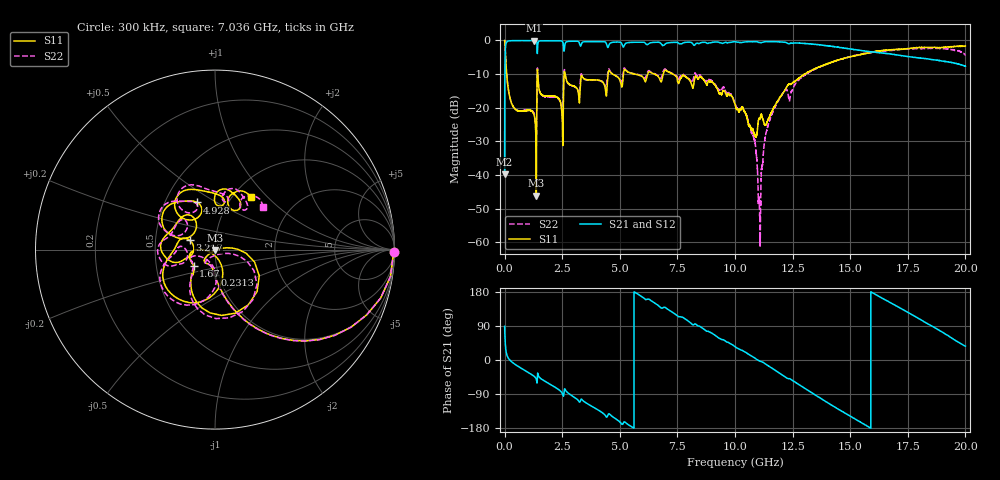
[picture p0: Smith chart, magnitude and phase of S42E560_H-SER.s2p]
!{S42E560}
!Johanson Technology Inc.
!www.johansontechnology.com
!Test Board Conditions:
!Substrate Type  RO4350B
!Substrate Thickness  50 mil
!Substrate Dk  3.66
!TL Type: GCPW
!TL Trace Width  60 mil
!TL Gap  10 mil
!Electrode orientation  Horizontal
!DUT TOPOLOGY	SERIES
!Mounting Pad LxW  14x55 mil
! Created Wed Nov 25 22:20:49 2020
# khz S ma R 50
! 2 Port Network Data from SP1.SP block
! freq  magS11  angS11  magS21  angS21  magS12  angS12  magS22  angS22
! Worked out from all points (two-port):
!   20001 points, 300 kHz to 20 GHz, reference 50 ohm
!   highest |S21| = -0.03 dB at 1.282 GHz (marker M1); lowest = -39.8 dB at 300 kHz (marker M2)
!   |S21| within 3 dB of the highest: 29.19 MHz to 1.413 GHz (1.384 GHz wide, 192 % of centre); 2.586 GHz to 15.52 GHz (12.93 GHz wide, 143 % of centre)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
!   lowest |S11| = -46.1 dB at 1.376 GHz (marker M3), VSWR 1.01, Z = 50.2 - j0.464 ohm
!   |S11| at or under -10 dB: 88.87 MHz to 1.415 GHz (1.326 GHz wide, 176 % of centre); 2.627 GHz to 4.492 GHz (1.865 GHz wide, 52.4 % of centre); 7.299 GHz to 13.01 GHz (5.716 GHz wide, 56.3 % of centre)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
!   |S22| runs from -61.2 to 0.0 dB; largest |S21 - S12| = 0.02
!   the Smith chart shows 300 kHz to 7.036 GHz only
!   S11 on the Smith chart (normalised r, x): 300 kHz: open; 231.3 MHz: 0.96, -0.27; 1.67 GHz: 0.77, -0.15; 3.217 GHz: 0.75, +0.08; 4.928 GHz: 0.72, +0.41; 7.036 GHz: 1.20, +0.80
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300  0.9955 -0.7  0.0102 88.8  0.01021 88.8  0.9951 -0.7
104300  0.2748 -77.8  0.9605 12.1  0.9601 12.1  0.2763 -78.2
231300  0.1404 -91.0  0.9882 -0.6  0.9881 -0.6  0.1413 -91.7
1282300  0.07769 -137.7  0.996 -43.2  0.9953 -43.2  0.07996 -128.4
1376300  0.00493 -69.7  0.9804 -51.0  0.9812 -50.9  0.03055 -62.2
1670300  0.1514 -141.9  0.9866 -53.1  0.9874 -53.1  0.1494 -143.9
3217300  0.1507 159.8  0.9596 -108.2  0.959 -108.2  0.163 179.9
3334300  0.3034 177.0  0.8873 -103.2  0.8859 -103.3  0.3184 178.7
4928300  0.2809 110.7  0.9472 -159.8  0.9464 -159.8  0.2834 112.7
6667300  0.2902 60.3  0.9388 143.9  0.9373 143.9  0.2975 52.6
7036300  0.3526 55.7  0.9111 135.8  0.9108 135.8  0.3579 41.7
8611300  0.2689 -9.8  0.9364 83.1  0.9354 83.2  0.2735 -2.5
1.00003e7  0.1124 -42.4  0.9567 35.3  0.9569 35.3  0.1171 -62.8
1.08033e7  0.04331 -7.1  0.9579 7.3  0.958 7.3  0.03696 -128.4
1.10723e7  0.06934 31.5  0.9341 -2.6  0.9337 -2.5  0.002574 -120.2
1.13253e7  0.0554 36.5  0.9605 -10.6  0.9597 -10.5  0.03882 120.7
1.16353e7  0.09303 58.9  0.9601 -22.8  0.959 -22.8  0.08597 70.9
1.33343e7  0.3589 14.2  0.8808 -86.5  0.8836 -86.3  0.3545 -5.8
1.49913e7  0.5707 -53.7  0.7492 -147.8  0.7461 -148.1  0.5716 -61.5
1.66673e7  0.7182 -107.1  0.6364 154.1  0.6197 154.2  0.7057 -122.5
1.86233e7  0.7877 -171.8  0.5157 86.9  0.5192 87.2  0.7595 173.4
2e7  0.827 142.7  0.413 36.5  0.4164 37.3  0.6055 111.2
